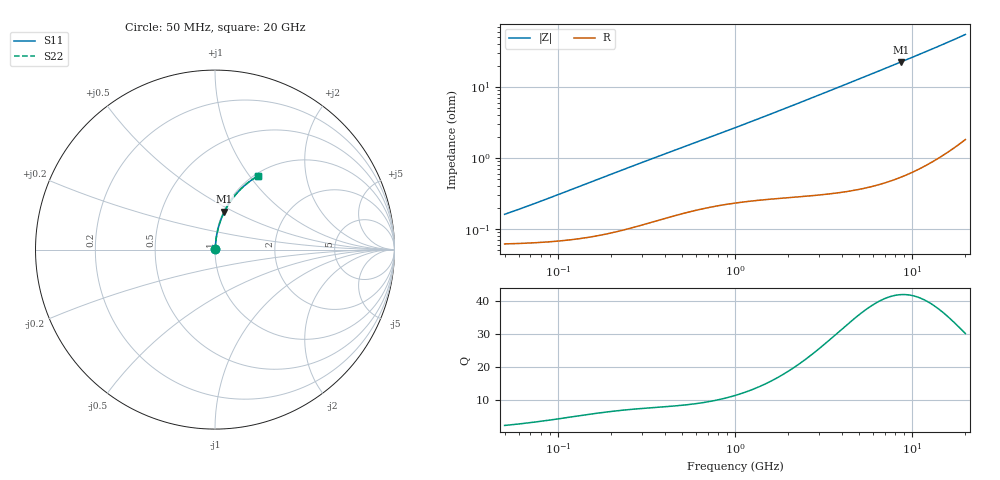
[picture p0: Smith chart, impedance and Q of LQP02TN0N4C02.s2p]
!Murata Part Number: LQP02TN0N4C02
!These Parameters are Measured in Series Mode Connection
!  o--[Z]--o
!Port1  Port2
!  o-------o
!Freq. Start=50[MHz] Stop=20[GHz], 401[Steps]
# Hz S RI R 50
!Freq.(Hz) S11(Real) S11(Imag) S21(Real) S21(Imag) S12(Real) S12(Imag) S22(Real) S22(Imag)
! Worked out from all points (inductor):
!   401 points, 50 MHz to 20 GHz, reference 50 ohm
!   read as one part in series: L = 473 pH near 63.54 MHz
!   highest Q = 41.9 at 8.645 GHz (marker M1), where L = 413 pH
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5e7  0.000619 0.00149  0.9994 -0.00149  0.9994 -0.00149  0.000619 0.00149
5.229804e7  0.000621 0.00155  0.9994 -0.00155  0.9994 -0.00155  0.000621 0.00155
7.056486e7  0.000641 0.00209  0.9994 -0.00209  0.9994 -0.00209  0.000641 0.00209
1.364002e8  0.000755 0.00402  0.9992 -0.00402  0.9992 -0.00402  0.000755 0.00402
2.409965e8  0.00103 0.00698  0.999 -0.00698  0.999 -0.00698  0.00103 0.00698
3.721004e8  0.00144 0.0105  0.9986 -0.0105  0.9986 -0.0105  0.00144 0.0105
6.380365e8  0.00219 0.0173  0.9978 -0.0173  0.9978 -0.0173  0.00219 0.0173
1e9  0.00301 0.0264  0.997 -0.0264  0.997 -0.0264  0.00301 0.0264
1.714689e9  0.00464 0.0443  0.9954 -0.0443  0.9954 -0.0443  0.00464 0.0443
2.728004e9  0.00783 0.0697  0.9922 -0.0697  0.9922 -0.0697  0.00783 0.0697
3.626126e9  0.0117 0.092  0.9883 -0.092  0.9883 -0.092  0.0117 0.092
4.677679e9  0.0177 0.118  0.9823 -0.118  0.9823 -0.118  0.0177 0.118
5.944466e9  0.0267 0.1487  0.9733 -0.1487  0.9733 -0.1487  0.0267 0.1487
7.442007e9  0.0399 0.184  0.9601 -0.184  0.9601 -0.184  0.0399 0.184
8.644534e9  0.0525 0.2114  0.9475 -0.2114  0.9475 -0.2114  0.0525 0.2114
1.098561e10  0.0816 0.2619  0.9184 -0.2619  0.9184 -0.2619  0.0816 0.2619
1.220001e10  0.099 0.2863  0.901 -0.2863  0.901 -0.2863  0.099 0.2863
1.354865e10  0.1198 0.312  0.8802 -0.312  0.8802 -0.312  0.1198 0.312
1.621653e10  0.1655 0.3576  0.8345 -0.3576  0.8345 -0.3576  0.1655 0.3576
1.774144e10  0.1938 0.3804  0.8062 -0.3804  0.8062 -0.3804  0.1938 0.3804
1.940974e10  0.2263 0.4025  0.7737 -0.4025  0.7737 -0.4025  0.2263 0.4025
2e10  0.2381 0.4096  0.7619 -0.4096  0.7619 -0.4096  0.2381 0.4096
